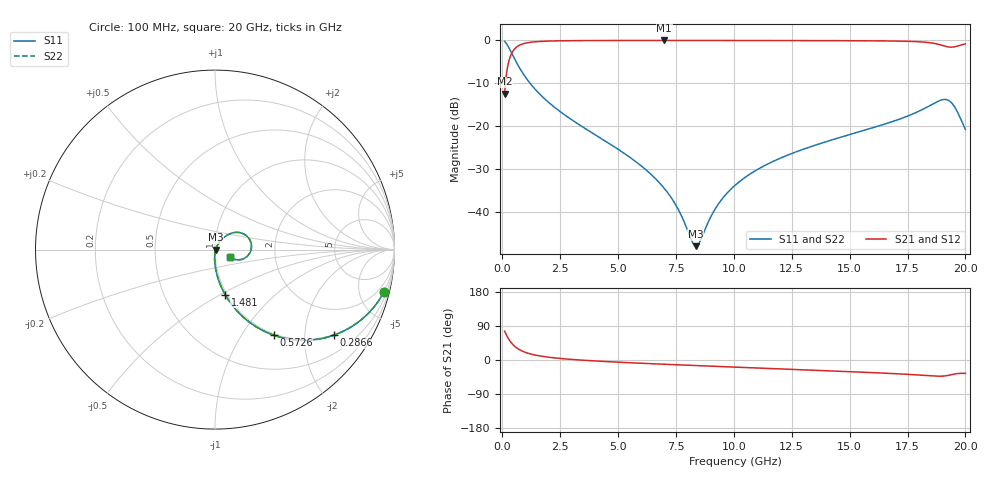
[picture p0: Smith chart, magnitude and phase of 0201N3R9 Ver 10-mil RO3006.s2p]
# GHz S MA R 50
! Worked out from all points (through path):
!   1601 points, 100 MHz to 20 GHz, reference 50 ohm
!   highest |S21| = -0.03 dB at 6.99 GHz (marker M1); lowest = -12.5 dB at 100 MHz (marker M2)
!   group delay of S21, straight-line fit = 8.65 ps
!   lowest |S11| = -48.0 dB at 8.358 GHz (marker M3), VSWR 1.01, Z = 50.4 - j0.116 ohm
!   |S11| at or under -10 dB: 1.197 GHz to end of sweep
!   |S22| runs from -48.0 to -0.3 dB; largest |S21 - S12| = 0
!   S11 on the Smith chart (normalised r, x): 100 MHz: 0.98, -8.05; 286.6 MHz: 0.98, -2.80; 572.6 MHz: 0.98, -1.40; 1.481 GHz: 0.98, -0.53; 20 GHz: 1.18, -0.09
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0.1  0.9711 -14.0  0.2384 76.0  0.2384 76.0  0.9711 -14.0
0.2865625  0.8172 -35.6  0.5755 54.3  0.5755 54.3  0.8172 -35.6
0.572625  0.5774 -55.6  0.8152 34.3  0.8152 34.3  0.5774 -55.6
0.9333125  0.3956 -68.1  0.9169 21.7  0.9169 21.7  0.3956 -68.1
1.480563  0.2576 -77.3  0.9643 12.3  0.9643 12.3  0.2576 -77.3
3.420812  0.09969 -88.8  0.9923 -0.3  0.9923 -0.3  0.09969 -88.8
5.560062  0.04224 -92.9  0.9957 -7.4  0.9957 -7.4  0.04224 -92.9
6.741625  0.02247 -91.4  0.996 -10.6  0.996 -10.6  0.02247 -91.4
6.990375  0.01885 -90.1  0.996 -11.2  0.996 -11.2  0.01885 -90.1
7.550063  0.01129 -83.1  0.996 -12.7  0.996 -12.7  0.01129 -83.1
8.196813  0.004499 -43.3  0.9959 -14.3  0.9959 -14.3  0.004499 -43.3
8.3585  0.003977 -16.8  0.9958 -14.7  0.9958 -14.7  0.003977 -16.8
8.520188  0.004423 9.8  0.9958 -15.1  0.9958 -15.1  0.004423 9.8
9.266438  0.01161 51.9  0.9955 -16.9  0.9955 -16.9  0.01161 51.9
10.05  0.02036 58.8  0.9952 -18.8  0.9952 -18.8  0.02036 58.8
11.39325  0.03533 60.3  0.9943 -22.0  0.9943 -22.0  0.03533 60.3
13.37081  0.05813 57.9  0.9924 -26.7  0.9924 -26.7  0.05813 57.9
16.69162  0.1092 49.1  0.9828 -35.2  0.9828 -35.2  0.1092 49.1
18.44531  0.1721 32.7  0.9388 -41.5  0.9388 -41.5  0.1721 32.7
19.12937  0.2044 6.8  0.8527 -41.9  0.8527 -41.9  0.2044 6.8
19.49006  0.1745 -15.2  0.8358 -37.5  0.8358 -37.5  0.1745 -15.2
20  0.09147 -26.0  0.9092 -35.4  0.9092 -35.4  0.09147 -26.0
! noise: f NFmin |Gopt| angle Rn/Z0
0.1  0.0006975  0.9392  0.643  0.002563
2.301  0.004564  0.7986  4.301  0.004687
4.515  0.007323  0.7594  8.102  0.006135
6.729  0.00976  0.7352  11.9  0.007288
8.943  0.01206  0.7189  15.68  0.00834
11.14  0.01439  0.709  19.4  0.009459
13.36  0.01709  0.708  23.12  0.01106
15.57  0.0216  0.7288  26.84  0.01501
17.79  0.03911  0.8209  30.67  0.0426
20  0.08623  0.905  34.52  0.1815
